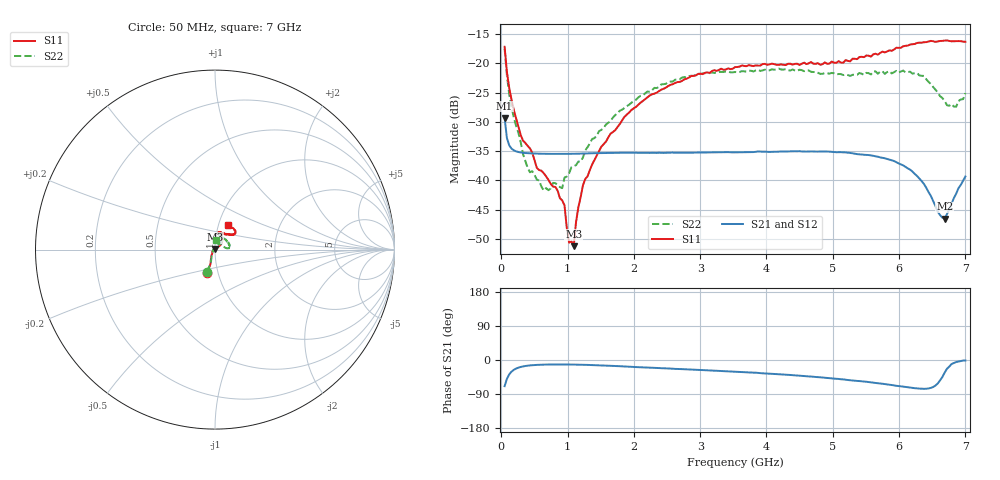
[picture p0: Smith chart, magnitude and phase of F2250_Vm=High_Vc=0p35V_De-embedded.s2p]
! Integrated Device Technology
! Corporate Headquarters
! 6024 Silver Creek Valley Road
! San Jose, CA 95138  USA
! Phone:  1-408-284-8200
! Toll Free:  1-800-223-1366
! Webpage:  http://www.idt.com/
! Timing and RF Division
! 515 Groton Road, Suite 102
! Westford, MA 01886-6024
! Device:  F2250
! Description: Voltage Variable RF Attenuator
! Frequency:  50.0 -  6000.00 MHz
! Package:  3x3 mm Thin QFN Plastic Package: 16 pin
! Ports:  2 RF, 3 DC
!  Pin  1  = GND
!  Pin  2  = NC
!  Pin  3  = RF1  = Port 1
!  Pin  4  = NC
!  Pin  5  = GND
!  Pin  6  = GND
!  Pin  7  = GND
!  Pin  8  = GND
!  Pin  9  = NC
!  Pin 10  = RF2  = Port 2
!  Pin 11  = NC
!  Pin 12  = GND
!  Pin 13  = GND
!  Pin 14  = VCNTRL
!  Pin 15  = VDD
!  Pin 16  = VMODE
! Vcntrl:  0.350 Volts
! Vmode:  +3.300 Volts
! Vdd:  +3.30  Volts
! Current:  1.257 mA
! Data:  The device was measured on a the F2250 evaluation board which has
!  individual transmission lines to the RF pins.  Data was collected
!  using a calibrated network analyzer.  The evaluation board was
!  de-embedded using a TRL calibration technique.
!  The reference plane is the edge of the package pin.
! Misc:  SN 10
!  Action Tracker AT0258
! Date Measured:  2014-11-26
! Date:  2015-10-15  MJV
! Note:
!  Integrated Device Technology supplies this data as a sample of measured
!  data at the package pin for this product.  Your particular data for this
!  product may vary.
!  Data was taken at 25 degrees C.
!  Integrated Device Technology reserves the right to change this data at anytime.
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# GHz S dB R 50
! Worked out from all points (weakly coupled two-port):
!   201 points, 50 MHz to 7 GHz, reference 50 ohm
!   highest |S21| = -29.34 dB at 50 MHz (marker M1); lowest = -46.6 dB at 6.687 GHz (marker M2)
!   lowest |S11| = -51.3 dB at 1.093 GHz (marker M3), VSWR 1.01, Z = 50 + j0.274 ohm
!   |S11| at or under -10 dB: start of sweep to end of sweep
!   |S22| runs from -41.7 to -17.5 dB; largest |S21 - S12| = 5e-05
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0.05  -17.18 -108.5  -29.34 -69.0  -29.34 -69.0  -17.52 -109.8
0.08475  -21.47 -107.4  -32.79 -49.7  -32.78 -49.7  -22.09 -107.3
0.189  -28.00 -120.0  -34.87 -25.9  -34.87 -25.9  -29.30 -120.3
0.328  -33.23 -134.1  -35.30 -16.9  -35.30 -16.9  -35.50 -134.7
0.43225  -34.54 -145.3  -35.39 -14.2  -35.39 -14.2  -38.63 -163.1
0.5365  -37.89 -154.7  -35.43 -12.9  -35.44 -12.9  -39.89 -178.1
0.71025  -39.91 -167.5  -35.48 -12.0  -35.47 -12.0  -41.69 146.5
0.91875  -43.44 155.8  -35.49 -11.8  -35.49 -11.8  -41.34 114.5
0.9535  -44.28 171.1  -35.49 -11.9  -35.49 -11.9  -39.52 112.6
1.023  -50.66 140.1  -35.48 -12.0  -35.48 -12.0  -38.80 94.4
1.0925  -51.25 90.1  -35.46 -12.1  -35.46 -12.1  -37.56 86.0
1.12725  -47.14 61.2  -35.45 -12.2  -35.45 -12.2  -37.41 78.5
1.2315  -40.85 40.7  -35.41 -12.6  -35.42 -12.6  -36.11 65.3
1.6485  -32.02 41.1  -35.33 -15.3  -35.33 -15.3  -29.86 54.2
2.37825  -24.75 46.6  -35.29 -21.2  -35.29 -21.2  -24.06 51.0
3.525  -20.65 71.7  -35.22 -30.9  -35.23 -31.0  -21.49 71.5
4.7065  -20.06 72.0  -35.06 -44.3  -35.07 -44.3  -21.50 69.5
5.85325  -17.79 40.5  -36.48 -65.2  -36.48 -65.2  -21.34 22.0
6.3745  -16.40 41.0  -40.62 -76.1  -40.63 -76.1  -22.16 5.8
6.68725  -16.11 47.9  -46.56 -33.3  -46.55 -32.9  -26.42 27.2
6.861  -16.22 54.5  -42.28 -5.3  -42.25 -5.4  -27.42 57.7
7  -16.32 62.4  -39.35 -1.4  -39.32 -1.6  -25.11 84.9
